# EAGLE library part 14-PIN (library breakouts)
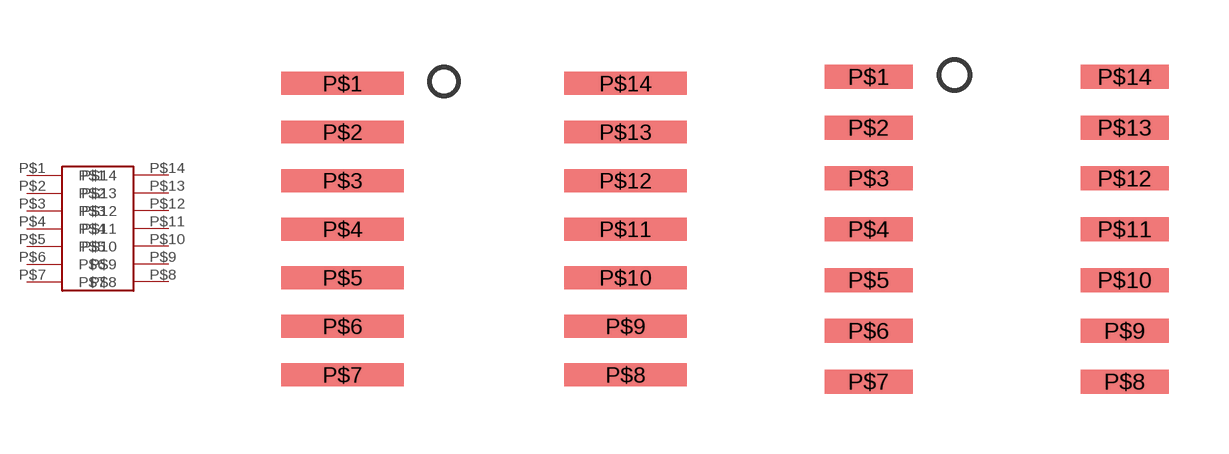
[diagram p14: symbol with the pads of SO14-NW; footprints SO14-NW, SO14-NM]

Designator prefix -

## 14-PINSOIC-NW  [SO14-NW]
P$1  P$1
P$2  P$2
P$3  P$3
P$4  P$4
P$5  P$5
P$6  P$6
P$7  P$7
P$8  P$8
P$9  P$9
P$10  P$10
P$11  P$11
P$12  P$12
P$13  P$13
P$14  P$14

## 14-PINSOIC-NM  [SO14-NM]
Pads as for SO14-NW

## 14-PINSOIC-M  [SO14-M]
Pads as for SO14-NW

## 14-PINSOIC-N  [SO14-N]
Pads as for SO14-NW

## 14-PINSOIC-MW  [SO14-MW]
Pads as for SO14-NW

## 14-PINSOIC-W  [SO14-W]
Pads as for SO14-NW

## 14-PINTSSOP-N  [TSSOP14-3.9]
Pads as for SO14-NW

## 14-PINTSSOP-W  [TSSOP14-5.3]
Pads as for SO14-NW

## 14-PINTSSOP-NW  [TSSOP14-NW]
Pads as for SO14-NW

## Footprint SO14-NW (pad centres in mm)
smd 3.2 x 0.6: P$1 -3.7,3.81; P$2 -3.7,2.54; P$3 -3.7,1.27; P$4 -3.7,0; P$5 -3.7,-1.27; P$6 -3.7,-2.54; P$7 -3.7,-3.81; P$8 3.7,-3.81; P$9 3.7,-2.54; P$10 3.7,-1.27; P$11 3.7,0; P$12 3.7,1.27; P$13 3.7,2.54; P$14 3.7,3.81

## Footprint SO14-NM (pad centres in mm)
smd 2.2 x 0.6: P$1 -3.2,3.81; P$2 -3.2,2.54; P$3 -3.2,1.27; P$4 -3.2,0; P$5 -3.2,-1.27; P$6 -3.2,-2.54; P$7 -3.2,-3.81; P$8 3.2,-3.81; P$9 3.2,-2.54; P$10 3.2,-1.27; P$11 3.2,0; P$12 3.2,1.27; P$13 3.2,2.54; P$14 3.2,3.81

## Footprint SO14-M (pad centres in mm)
smd 1.2 x 0.6: P$1 -3.7,3.81; P$2 -3.7,2.54; P$3 -3.7,1.27; P$4 -3.7,0; P$5 -3.7,-1.27; P$6 -3.7,-2.54; P$7 -3.7,-3.81; P$8 3.7,-3.81; P$9 3.7,-2.54; P$10 3.7,-1.27; P$11 3.7,0; P$12 3.7,1.27; P$13 3.7,2.54; P$14 3.7,3.81

## Footprint SO14-N (pad centres in mm)
smd 1.2 x 0.6: P$1 -2.7,3.81; P$2 -2.7,2.54; P$3 -2.7,1.27; P$4 -2.7,0; P$5 -2.7,-1.27; P$6 -2.7,-2.54; P$7 -2.7,-3.81; P$8 2.7,-3.81; P$9 2.7,-2.54; P$10 2.7,-1.27; P$11 2.7,0; P$12 2.7,1.27; P$13 2.7,2.54; P$14 2.7,3.81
